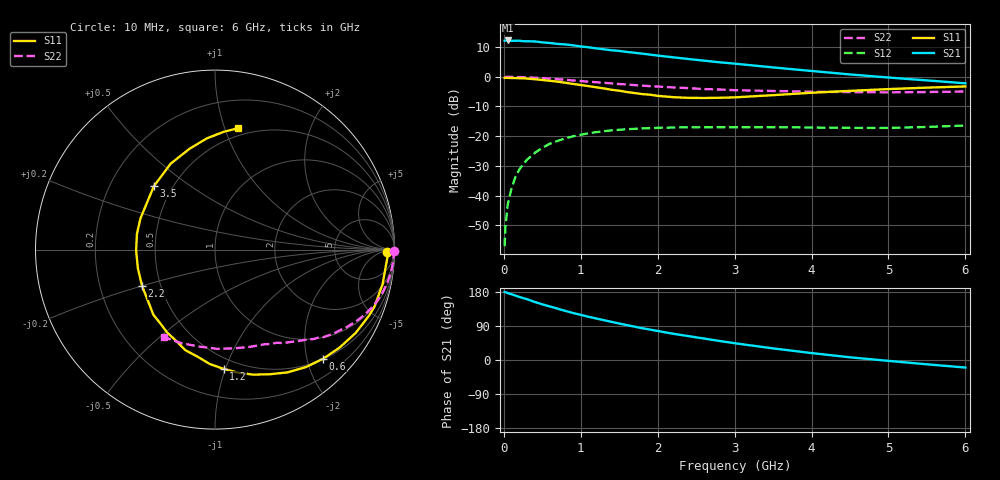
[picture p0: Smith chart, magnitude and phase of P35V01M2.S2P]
! SIEMENS Small Signal Semiconductors
! BFP181
! Si NPN RF Bipolar Junction Transistor in SOT143
! VCE = 5 V  IC = 1.2 mA
! Common Emitter S-Parameters:  March  1996
# GHz  S  MA  R  50
!  f  S11  S21  S12  S22
! GHz  MAG  ANG  MAG  ANG  MAG  ANG  MAG  ANG
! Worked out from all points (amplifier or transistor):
!   36 points, 10 MHz to 6 GHz, reference 50 ohm
!   highest |S21| = 12.3 dB at 50 MHz (marker M1)
!   |S21| within 3 dB of that: start of sweep to 1.304 GHz
!   unconditionally stable (mu >= 1): 2.973 GHz to end of sweep
!   at 250 MHz: K = 0.09, MSG = 20.8 dB, |S12| = -29.5 dB
!   at 1.4 GHz: K = 0.52, MSG = 13.5 dB, |S12| = -18.0 dB
!   at 6 GHz: K = 1.23, MAG = 4.2 dB, |S12| = -16.4 dB
!   S11 on the Smith chart (normalised r, x): 10 MHz: 43, -14; 600 MHz: 0.51, -2.31; 1.2 GHz: 0.41, -0.99; 2.2 GHz: 0.39, -0.20; 3.5 GHz: 0.40, +0.37; 6 GHz: 0.43, +1.11
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0.01  0.9591 -0.8  4.054 179.5  0.0014 92.0  0.9973 -0.3
0.02  0.9637 -1.6  4.066 179.2  0.0029 94.4  0.9905 -0.7
0.05  0.9593 -3.7  4.099 176.6  0.007 91.4  0.9967 -1.8
0.1  0.9539 -7.8  4.034 173.4  0.0132 84.0  0.9951 -3.6
0.2  0.9467 -15.2  4.064 166.5  0.0272 79.8  0.989 -7.2
0.3  0.9341 -23.1  3.977 160.6  0.0399 75.5  0.978 -10.7
0.4  0.9112 -30.6  3.946 153.3  0.052 70.2  0.9653 -14.1
0.6  0.8562 -45.2  3.713 141.2  0.0747 61.1  0.9319 -20.3
0.8  0.7941 -59.5  3.515 129.5  0.092 53.0  0.891 -25.8
0.9  0.7584 -66.3  3.396 124.0  0.0994 49.0  0.868 -28.5
1.1  0.6967 -79.6  3.149 114.1  0.112 42.3  0.8278 -32.9
1.2  0.6661 -85.9  3.015 109.6  0.1168 39.0  0.8106 -35.2
1.5  0.584 -106.5  2.732 96.2  0.128 31.4  0.7555 -40.5
1.7  0.5329 -120.1  2.543 87.9  0.1327 27.1  0.7237 -43.8
1.9  0.4998 -133.4  2.367 80.3  0.1364 23.1  0.6963 -46.7
2.2  0.4541 -153.5  2.132 69.3  0.1399 18.4  0.6631 -51.0
2.8  0.4435 168.6  1.758 50.3  0.1418 11.2  0.6108 -59.4
3.5  0.4908 133.9  1.44 30.6  0.1417 6.0  0.5767 -69.8
4  0.5386 117.3  1.254 18.3  0.1398 3.6  0.5606 -78.8
4.5  0.5798 104.1  1.097 7.1  0.138 2.4  0.5532 -88.7
5.5  0.6575 85.9  0.87 -11.4  0.143 4.2  0.554 -109.6
6  0.6884 79.3  0.777 -19.9  0.1512 4.1  0.5653 -120.5
